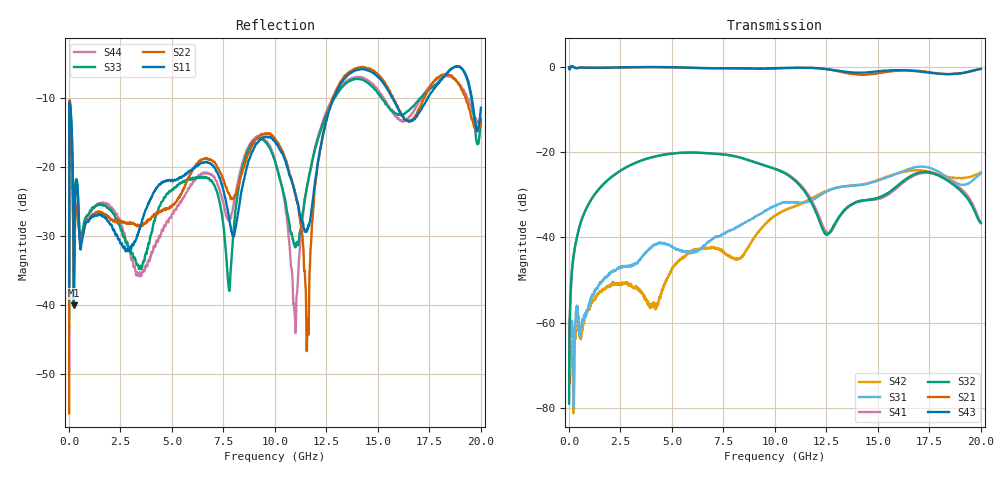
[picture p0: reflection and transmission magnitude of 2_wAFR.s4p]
!Keysight Technologies,N5225A,MY51451420,A.10.40.12
!Date: Tuesday, October 13, 2015 10:34:12
!Correction: S11(Full 4 Port(1,2,3,4))
!S12(Full 4 Port(1,2,3,4))
!S13(Full 4 Port(1,2,3,4))
!S14(Full 4 Port(1,2,3,4))
!S21(Full 4 Port(1,2,3,4))
!S22(Full 4 Port(1,2,3,4))
!S23(Full 4 Port(1,2,3,4))
!S24(Full 4 Port(1,2,3,4))
!S31(Full 4 Port(1,2,3,4))
!S32(Full 4 Port(1,2,3,4))
!S33(Full 4 Port(1,2,3,4))
!S34(Full 4 Port(1,2,3,4))
!S41(Full 4 Port(1,2,3,4))
!S42(Full 4 Port(1,2,3,4))
!S43(Full 4 Port(1,2,3,4))
!S44(Full 4 Port(1,2,3,4))
!S4P File: Measurements: <S11,S12,S13,S14>,
!<S21,S22,S23,S24>,
!<S31,S32,S33,S34>,
!<S41,S42,S43,S44>:
# Hz S  dB  R 50
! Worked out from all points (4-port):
!   2000 points, 10 MHz to 20 GHz, reference 50 ohm
!   strongest paths, dB at 10 MHz, 5.01 GHz, 10.01 GHz, 15.01 GHz, 20 GHz:
!     S43: -0.1, -0.1, -0.3, -1.0, -0.5
!     S21: -0.1, -0.1, -0.4, -1.5, -0.5
!     S32: -79.0, -20.3, -24.0, -30.7, -36.6
!     S41: -59.3, -20.3, -23.9, -31.0, -36.6
!     S31: -70.6, -42.2, -32.5, -26.7, -25.0
!     S42: -73.3, -47.4, -34.9, -26.5, -24.7
!   lowest |S11| = -40.0 dB at 240 MHz (marker M1), VSWR 1.02, Z = 50.5 - j0.872 ohm
!   |S11| at or under -10 dB: start of sweep to 12.85 GHz; 15.71 GHz to 17.42 GHz (1.718 GHz wide, 10.4 % of centre); 19.56 GHz to end of sweep
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1e7  -39.19 -16.0  -0.06 0.4  -63.14 -91.8  -63.48 59.5
     -0.06 0.4  -55.69 119.8  -63.72 56.9  -66.95 131.4
     -70.64 54.8  -79.00 87.3  -36.90 -8.6  -0.10 0.6
     -59.33 109.2  -73.34 -126.2  -0.10 0.1  -49.59 0.4
2.4e8  -40.05 -60.3  -0.08 0.2  -84.33 -59.1  -44.00 89.9
       -0.08 0.2  -35.53 4.1  -44.01 89.6  -79.32 103.0
       -80.00 97.1  -43.78 89.8  -40.21 -49.8  -0.11 0.1
       -44.00 90.0  -77.56 111.2  -0.09 0.1  -35.04 10.8
5.24e9  -21.78 -65.7  -0.14 3.1  -42.86 2.6  -20.23 92.0
        -0.14 3.2  -24.86 -135.6  -20.22 93.1  -45.93 -52.8
        -42.87 3.0  -20.22 93.0  -22.75 -66.4  -0.12 1.7
        -20.23 92.2  -46.01 -52.9  -0.11 1.7  -25.86 -138.1
9.84e9  -15.83 28.0  -0.41 -7.6  -32.93 77.7  -23.65 84.3
        -0.41 -7.3  -15.44 137.2  -23.67 84.7  -35.52 152.5
        -32.97 78.0  -23.69 84.6  -17.87 31.9  -0.34 -10.1
        -23.63 84.6  -35.52 152.2  -0.33 -10.0  -17.53 129.0
1.157e10  -28.86 -42.2  -0.23 -6.6  -31.67 -0.9  -29.64 85.4
          -0.23 -6.3  -43.96 -159.4  -30.09 86.0  -31.41 173.9
          -31.68 -0.4  -30.13 86.0  -22.65 27.4  -0.22 -9.8
          -29.63 85.7  -31.39 174.0  -0.21 -9.6  -22.79 104.5
1.342e10  -7.09 -48.5  -1.40 -5.3  -28.04 -53.6  -33.49 -164.4
          -1.40 -4.9  -6.78 -145.3  -33.49 -161.2  -28.01 -148.9
          -28.02 -53.3  -33.50 -161.2  -7.97 -47.9  -1.15 -7.5
          -33.51 -163.6  -27.99 -148.6  -1.14 -7.2  -7.77 -149.1
2e10  -11.43 -89.7  -0.48 -20.4  -24.99 145.4  -36.60 -102.6
      -0.48 -19.9  -13.65 -61.3  -36.56 -91.9  -24.75 0.5
      -25.00 145.7  -36.63 -92.1  -13.12 -89.6  -0.49 -24.8
      -36.59 -102.2  -24.75 0.4  -0.47 -24.6  -13.05 -46.1
